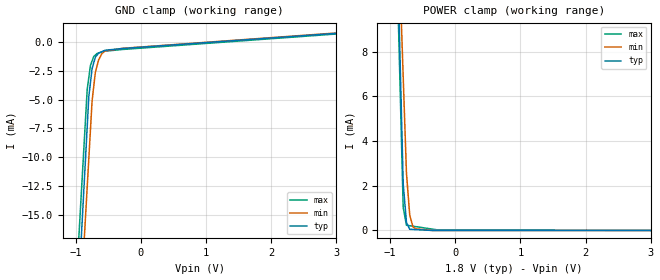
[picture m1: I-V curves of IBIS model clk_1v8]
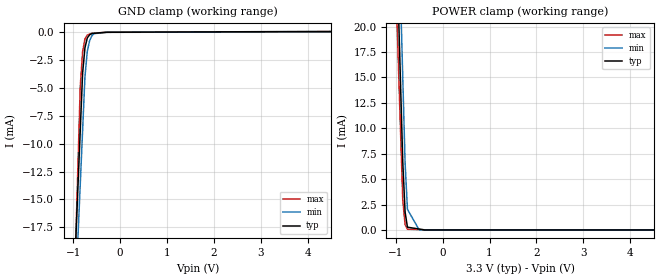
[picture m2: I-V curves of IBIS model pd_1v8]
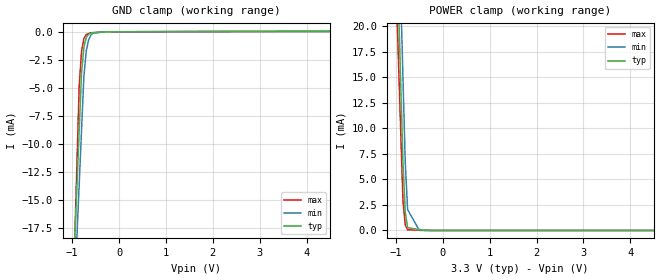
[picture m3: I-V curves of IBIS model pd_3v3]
[IBIS Ver]   3.2
[Comment Char] |_char
[File Name]   dac5688.ibs
[File Rev]   3.1
[Source]
| This model file was created by Teraspeed Consulting Group LLC
| (http://www.teraspeed.com/).
[Date]   07-02-2008
[Notes]   Quality Check of this IBIS model: Model Passes IBIS Check
   Model parses into ICX IS. Simulation done with Hyperlynx.
   1. MIN TYP MAX information is based on Temprature and Voltage
   characteristics only.
[Disclaimer]
| This model is designed as an aid for customers of Texas Instruments.
| TI and its licensors and suppliers make no warranties, either expressed
| or implied, with respect to this  model, including the warranties of
| merchantability or fitness for a particular purpose.
| The model is provided solely on an "as is" basis. The entire risk as to
| its quality and performance is with the customer.
[Copyright]
| (C) Copyright 2008 Texas Instruments Incorporated. All rights reserved.
[Component]   DAC5688
[Manufacturer] TI
[Package]
| variable   typ   min   max
R_pkg  1.5243E-02  1.4866E-02  1.5620E-02
L_pkg  1.8292E-09  1.7839E-09  1.8745E-09
C_pkg  5.0811E-13  4.9554E-13  5.2068E-13
[Pin] signal_name  model_name  R_pin  L_pin C_pin
1   CLKVDD   POWER   2.060E-02   1.850E-09   5.150E-13
2   CLK2   clk_1v8   1.970E-02   1.780E-09   4.930E-13
3   CLK2C   clk_1v8   1.890E-02   1.700E-09   4.720E-13
4   GND   GND   1.800E-02   1.620E-09   4.510E-13
5   SYNC   in_pd   1.720E-02   1.550E-09   4.300E-13
6   TXENABLE   in_pd   1.640E-02   1.480E-09   4.100E-13
7   DA15   in_pd   1.560E-02   1.410E-09   3.910E-13
8   DA14   in_pd   1.490E-02   1.340E-09   3.720E-13
9   IOVDD   POWER   1.490E-02   1.340E-09   3.720E-13
10   DVDD   POWER   1.560E-02   1.410E-09   3.910E-13
11   DA13   in_pd   1.640E-02   1.480E-09   4.100E-13
12   DA12   in_pd   1.720E-02   1.550E-09   4.300E-13
13   DA11   in_pd   1.800E-02   1.620E-09   4.510E-13
14   DA10   in_pd   1.890E-02   1.700E-09   4.720E-13
15   DA9   in_pd   1.970E-02   1.780E-09   4.930E-13
16   DA8   in_pd   2.060E-02   1.850E-09   5.150E-13
17   DA7   in_pd   2.060E-02   1.850E-09   5.150E-13
18   DA6   in_pd   1.970E-02   1.780E-09   4.930E-13
19   DA5   in_pd   1.890E-02   1.700E-09   4.720E-13
20   DA4   in_pd   1.800E-02   1.620E-09   4.510E-13
21   DA3   in_pd   1.720E-02   1.550E-09   4.300E-13
22   DA2   in_pd   1.640E-02   1.480E-09   4.100E-13
23   DA1   in_pd   1.560E-02   1.410E-09   3.910E-13
24   DA0   in_pd   1.490E-02   1.340E-09   3.720E-13
25   CLKO_CLK1   clk_io   1.490E-02   1.340E-09   3.720E-13
26   LOCK_CLK1C  clk_io   1.560E-02   1.410E-09   3.910E-13
27   DB0   in_pd   1.640E-02   1.480E-09   4.100E-13
28   DB1   in_pd   1.720E-02   1.550E-09   4.300E-13
29   DB2   in_pd   1.800E-02   1.620E-09   4.510E-13
30   DB3   in_pd   1.890E-02   1.700E-09   4.720E-13
31   DB4   in_pd   1.970E-02   1.780E-09   4.930E-13
32   DB5   in_pd   2.060E-02   1.850E-09   5.150E-13
33   DB6   in_pd   2.060E-02   1.850E-09   5.150E-13
34   DB7   in_pd   1.970E-02   1.780E-09   4.930E-13
35   DB8   in_pd   1.890E-02   1.700E-09   4.720E-13
36   DB9   in_pd   1.800E-02   1.620E-09   4.510E-13
37   DB10   in_pd   1.720E-02   1.550E-09   4.300E-13
38   DB11   in_pd   1.640E-02   1.480E-09   4.100E-13
39   DVDD   POWER   1.560E-02   1.410E-09   3.910E-13
40   DB12   in_pd   1.490E-02   1.340E-09   3.720E-13
41   DB13   in_pd   1.490E-02   1.340E-09   3.720E-13
42   DB14   in_pd   1.560E-02   1.410E-09   3.910E-13
43   DB15   in_pd   1.640E-02   1.480E-09   4.100E-13
44   VFUSE   POWER   1.720E-02   1.550E-09   4.300E-13
45   SDO   sif_tri   1.800E-02   1.620E-09   4.510E-13
46   SDIO   sif_io   1.890E-02   1.700E-09   4.720E-13
47   SCLK   in_pd   1.970E-02   1.780E-09   4.930E-13
48   _SDEN   in_pu   2.060E-02   1.850E-09   5.150E-13
49   _RESET   in_pu   2.060E-02   1.850E-09   5.150E-13
50   DVDD   POWER   1.970E-02   1.780E-09   4.930E-13
51   AVDD   POWER   1.890E-02   1.700E-09   4.720E-13
52   IOUTA1   analog   1.800E-02   1.620E-09   4.510E-13
53   IOUTA2   analog   1.720E-02   1.550E-09   4.300E-13
54   AVDD   POWER   1.640E-02   1.480E-09   4.100E-13
55   AVDD   POWER   1.560E-02   1.410E-09   3.910E-13
56   EXTIO   term   1.490E-02   1.340E-09   3.720E-13
57   BIASJ   term   1.490E-02   1.340E-09   3.720E-13
58   EXTLO   term   1.560E-02   1.410E-09   3.910E-13
59   AVDD   POWER   1.640E-02   1.480E-09   4.100E-13
60   IOUTB1   analog   1.720E-02   1.550E-09   4.300E-13
61   IOUTB2   analog   1.800E-02   1.620E-09   4.510E-13
62   AVDD   POWER   1.890E-02   1.700E-09   4.720E-13
63   DVDD   POWER   1.970E-02   1.780E-09   4.930E-13
64   LPF   term   2.060E-02   1.850E-09   5.150E-13
[Diff Pin] inv_pin vdiff tdelay_typ tdelay_min tdelay_max
|diff pair pins 25/26
|  Remove the comment character ( | ) when used with differential
|  input on CLKO_CLK1/LOCK_CLK1C
|25  26  500mV  NA  NA  NA
2   3   500mV  NA  NA  NA
52  53  NA  NA  NA  NA
61  60  NA  NA  NA  NA
[Model Selector]  in_pd
pd_1v8   pull dwn input w/1.8v thresholds
pd_3v3   pull dwn input w/3.3v thresholds
[Model Selector]  in_pu
pu_1v8   pull up input w/1.8v thresholds
pu_3v3   pull up input w/3.3v thresholds
[Model Selector]  sif_io
io_1v8   io w/1.8v input thresholds
io_3v3   io w/3.3v input thresholds
[Model Selector]  clk_io
io_1v8   io w/1.8v input thresholds
io_3v3   io w/1.8v input thresholds
[Model] analog
Model_type Terminator
C_comp   0  0  0
| variable   typ   min   max
[Voltage Range]   3.30000V  3.00000V  3.60000V
[POWER Clamp Reference]  3.30000V  3.00000V  3.60000V
[GND Clamp Reference]   0.00000V  0.00000V  0.00000V
[Temperature Range]   25   85   -40
[Model] term
Model_type Terminator
C_comp   0  0  0
| variable   typ   min   max
[Voltage Range]   3.30000V  3.00000V  3.60000V
[POWER Clamp Reference]  3.30000V  3.00000V  3.60000V
[GND Clamp Reference]   0.00000V  0.00000V  0.00000V
[Temperature Range]   25   85   -40
| Models and submodels in the file (10): clk_1v8 (Input), pd_1v8 (Input), pd_3v3 (Input), pu_1v8 (Input), pu_3v3 (Input), io_1v8 (I/O), io_3v3 (I/O), sif_tri (3-state), analog (Terminator), term (Terminator)
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[Model] clk_1v8
Model_type Input
Vinl = 540.000mV
Vinh = 1.25000V
C_comp 652.000fF 652.000fF 652.000fF
| variable typ   min   max
[Voltage Range] 1.80000V 1.71000V 2.15000V
[POWER Clamp Reference] 1.80000V 1.71000V 2.15000V
[GND Clamp Reference] 0.00000V 0.00000V 0.00000V
[Temperature Range]   25   85   -40
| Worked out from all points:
|   GND clamp passes 1 mA (typ) near -0.65 V on its own axis
|   POWER clamp passes 1 mA (typ) near -0.77 V on its own axis
[GND Clamp]
-1.8V     -110.5mA   -109.6mA   -101.3mA
-825mV    -7.382mA   -12.59mA   -4.131mA
-800mV    -4.738mA   -10.1mA    -3.09mA
-775mV    -3.532mA   -7.616mA   -2.049mA
-750mV    -2.326mA   -5.129mA   -1.669mA
-700mV    -1.345mA   -2.667mA   -1.158mA
-675mV    -1.168mA   -2.124mA   -1.026mA
-650mV    -991.3uA   -1.581mA   -978uA
-600mV    -865.1uA   -1.025mA   -881.1uA
-550mV    -739uA     -794.7uA   -818.8uA
-275mV    -585.3uA   -567.6uA   -669uA
3.6V      962.5uA    999.8uA    912.3uA
[POWER Clamp]
-1.8V     118.3mA    93.11mA    118.5mA
-1.125V   39.86mA    34.91mA    37.73mA
-800mV    2.087mA    6.885mA    1.031mA
-750mV    363uA      2.574mA    234.5uA
-700mV    54.12uA    695uA      212.7uA
-650mV    46.39uA    155.4uA    190.9uA
-600mV    38.66uA    71.83uA    169.1uA
-350mV    0A         0A         59.99uA
-275mV    0A         0A         27.27uA
3.6V      0A         0A         0A
[Model] pd_1v8
Model_type Input
Vinl = 0.54000V
Vinh = 1.25000V
C_comp 453.000fF 453.000fF 453.000fF
| variable typ   min   max
[Voltage Range] 3.30000V 3.00000V 3.60000V
[POWER Clamp Reference] 3.30000V 3.00000V 3.60000V
[GND Clamp Reference] 0.00000V 0.00000V 0.00000V
[Temperature Range]   25   85   -40
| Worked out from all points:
|   GND clamp passes 1 mA (typ) near -0.73 V on its own axis
|   POWER clamp passes 1 mA (typ) near -0.77 V on its own axis
[GND Clamp]
-3.3V     -260.8mA   -249.8mA   -357.6mA
-850mV    -8.825mA   -13.65mA   -4.88mA
-800mV    -3.684mA   -8.828mA   -1.762mA
-750mV    -1.397mA   -4.009mA   -603.5uA
-700mV    -515.7uA   -1.72mA    -250.5uA
-650mV    -229.7uA   -755.2uA   -171.2uA
-600mV    -117.4uA   -294.8uA   -91.99uA
-550mV    -98.6uA    -123.2uA   -77.84uA
-300mV    -4.599uA   -16.36uA   -7.124uA
-275mV    -4.2uA     -5.673uA   -6.948uA
6.6V      105.7uA    25.71uA    41.35uA
[POWER Clamp]
-3.3V     405mA      428.9mA    353.2mA
-1.05V    39.24mA    48.83mA    31.56mA
-850mV    6.729mA    15.05mA    2.968mA
-800mV    1.773mA    6.601mA    524.9uA
-750mV    272.7uA    2.03mA     68.76uA
-500mV    90.89uA    14.35uA    36.01uA
-450mV    54.54uA    0A         29.47uA
6.6V      0A         0A         0A
[Model] pd_3v3
Model_type Input
Vinl = 1.00000V
Vinh = 2.30000V
C_comp 453.000fF 453.000fF 453.000fF
| variable typ   min   max
[Voltage Range] 3.30000V 3.00000V 3.60000V
[POWER Clamp Reference] 3.30000V 3.00000V 3.60000V
[GND Clamp Reference] 0.00000V 0.00000V 0.00000V
[Temperature Range]   25   85   -40
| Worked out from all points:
|   GND clamp passes 1 mA (typ) near -0.73 V on its own axis
|   POWER clamp passes 1 mA (typ) near -0.77 V on its own axis
[GND Clamp]
-3.3V     -260.8mA   -249.8mA   -357.6mA
-850mV    -8.825mA   -13.65mA   -4.88mA
-800mV    -3.684mA   -8.828mA   -1.762mA
-750mV    -1.397mA   -4.009mA   -603.5uA
-700mV    -515.7uA   -1.72mA    -250.5uA
-650mV    -229.7uA   -755.2uA   -171.2uA
-600mV    -117.4uA   -294.8uA   -91.99uA
-550mV    -98.6uA    -123.2uA   -77.84uA
-300mV    -4.599uA   -16.36uA   -7.124uA
-275mV    -4.2uA     -5.673uA   -6.948uA
6.6V      105.7uA    25.71uA    41.35uA
[POWER Clamp]
-3.3V     405mA      428.9mA    353.2mA
-1.05V    39.24mA    48.83mA    31.56mA
-850mV    6.729mA    15.05mA    2.968mA
-800mV    1.773mA    6.601mA    524.9uA
-750mV    272.7uA    2.03mA     68.76uA
-500mV    90.89uA    14.35uA    36.01uA
-450mV    54.54uA    0A         29.47uA
6.6V      0A         0A         0A
